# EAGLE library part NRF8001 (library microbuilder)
nRF8001 - Bluetooth Low-Energy Transceiver VDD: 1.9-3.6V Temp: -40°C - 85°C
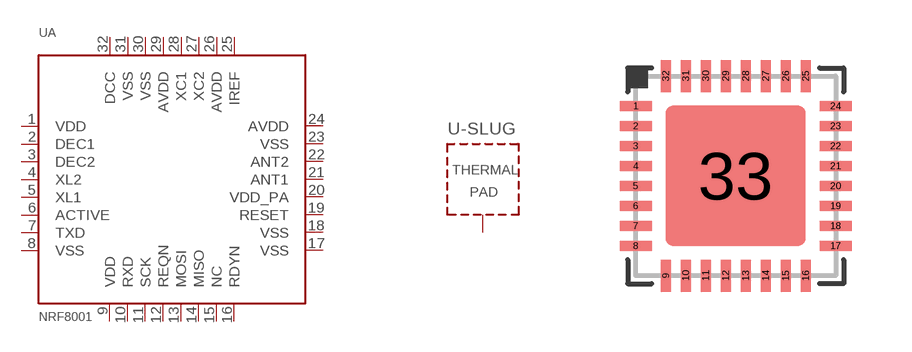
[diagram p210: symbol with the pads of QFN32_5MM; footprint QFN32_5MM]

Designator prefix U; gates A=NRF8001 -SLUG=THERMAL-SLUG

## NRF8001  [QFN32_5MM]
1  A:VDD  pwr
2  A:DEC1
3  A:DEC2
4  A:XL2  out
5  A:XL1  in
6  A:ACTIVE  out
7  A:TXD  out
8  A:VSS  pwr
9  A:VDD  pwr
10  A:RXD  in
11  A:SCK  in
12  A:REQN  in
13  A:MOSI  in
14  A:MISO  out
15  A:NC  nc
16  A:RDYN  out
17  A:VSS  pwr
18  A:VSS  pwr
19  A:RESET  in
20  A:VDD_PA
21  A:ANT1
22  A:ANT2
23  A:VSS  pwr
24  A:AVDD  pwr
25  A:IREF  out
26  A:AVDD  pwr
27  A:XC2  out
28  A:XC1  in
29  A:AVDD  pwr
30  A:VSS  pwr
31  A:VSS  pwr
32  A:DCC
33  -SLUG:TP  pwr

## Footprint QFN32_5MM (pad centres in mm)
QFN32 5x5mm 0.5mm pitch Source: Nordic nRF8001 Product Specification
smd 0.8 x 0.25: 1 -2.5,1.75; 2 -2.5,1.25; 3 -2.5,0.75; 4 -2.5,0.25; 5 -2.5,-0.25; 6 -2.5,-0.75; 7 -2.5,-1.25; 8 -2.5,-1.75; 17 2.5,-1.75; 18 2.5,-1.25; 19 2.5,-0.75; 20 2.5,-0.25; 21 2.5,0.25; 22 2.5,0.75; 23 2.5,1.25; 24 2.5,1.75
smd 0.25 x 0.8: 9 -1.75,-2.5; 10 -1.25,-2.5; 11 -0.75,-2.5; 12 -0.25,-2.5; 13 0.25,-2.5; 14 0.75,-2.5; 15 1.25,-2.5; 16 1.75,-2.5; 25 1.75,2.5; 26 1.25,2.5; 27 0.75,2.5; 28 0.25,2.5; 29 -0.25,2.5; 30 -0.75,2.5; 31 -1.25,2.5; 32 -1.75,2.5
smd 3.5 x 3.5: 33 0,0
